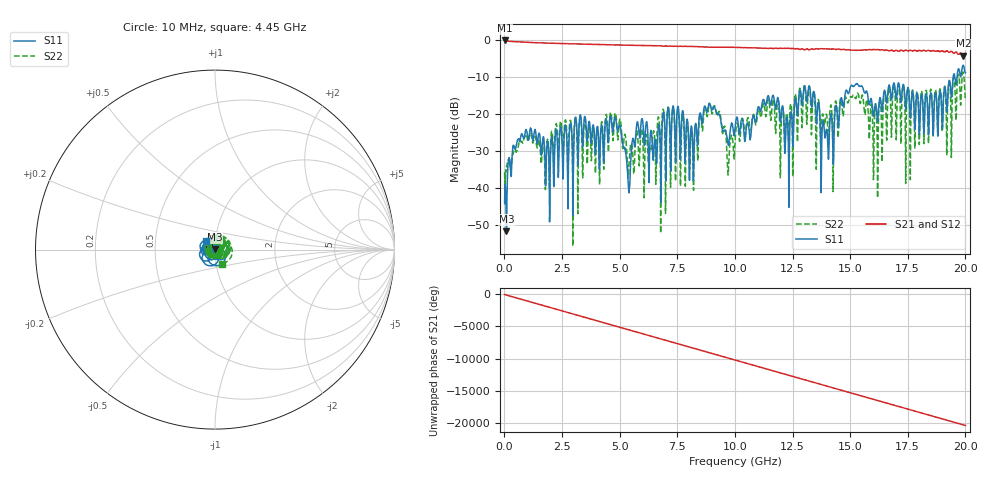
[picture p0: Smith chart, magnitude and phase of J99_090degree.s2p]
!Keysight Technologies,N5222A,MY51421036,A.10.65.16
!Date: Friday, March 31, 2023 15:04:34
!Correction: S11(Full 2 Port(1,2))
!S21(Full 2 Port(1,2))
!S12(Full 2 Port(1,2))
!S22(Full 2 Port(1,2))
!S2P File: Measurements: S11, S21, S12, S22:
# Hz S  dB  R 50
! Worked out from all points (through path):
!   2000 points, 10 MHz to 20 GHz, reference 50 ohm
!   highest |S21| = -0.04 dB at 10 MHz (marker M1); lowest = -4.1 dB at 19.91 GHz (marker M2)
!   group delay of S21, straight-line fit = 2.84 ns
!   lowest |S11| = -51.8 dB at 90 MHz (marker M3), VSWR 1.01, Z = 49.8 + j0.0643 ohm
!   |S11| at or under -10 dB: start of sweep to 19.47 GHz; 19.54432 GHz to 19.63788 GHz (93.56 MHz wide, 0.478 % of centre)
!   |S22| runs from -55.9 to -8.6 dB; largest |S21 - S12| = 0.019
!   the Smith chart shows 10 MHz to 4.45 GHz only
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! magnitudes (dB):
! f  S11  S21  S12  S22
! 10 MHz  -44.3  0.0  -0.1  -35.7
! 90 MHz  -51.8  -0.2  -0.2  -34.2
! 690 MHz  -26.6  -0.5  -0.4  -27.4
! 1.88 GHz  -27.6  -0.8  -0.8  -26.9
! 3.35 GHz  -23.2  -1.0  -1.0  -24.5
! 4.87 GHz  -23.3  -1.3  -1.2  -22.2
! 5.39 GHz  -40.2  -1.3  -1.3  -35.3
! 5.84 GHz  -25.2  -1.4  -1.4  -33.2
! 6.68 GHz  -23.6  -1.5  -1.5  -20.8
! 8.12 GHz  -23.3  -1.7  -1.7  -24.9
! 8.96 GHz  -18.3  -1.9  -1.9  -18.2
! 10.01 GHz  -23.6  -1.9  -1.9  -27.9
! 11.62 GHz  -15.3  -2.2  -2.2  -17.4
! 12.26 GHz  -20.8  -2.2  -2.2  -20.1
! 13.34 GHz  -18.0  -2.3  -2.3  -22.4
! 13.99 GHz  -24.5  -2.3  -2.3  -20.4
! 15.09 GHz  -12.3  -2.7  -2.6  -15.5
! 16.1 GHz  -17.2  -2.5  -2.5  -18.0
! 16.67 GHz  -12.5  -2.8  -2.8  -13.2
! 18.71 GHz  -14.2  -3.0  -2.8  -13.5
! 19.91 GHz  -6.8  -4.1  -3.9  -8.7
! 20 GHz  -8.8  -3.5  -3.4  -16.1
